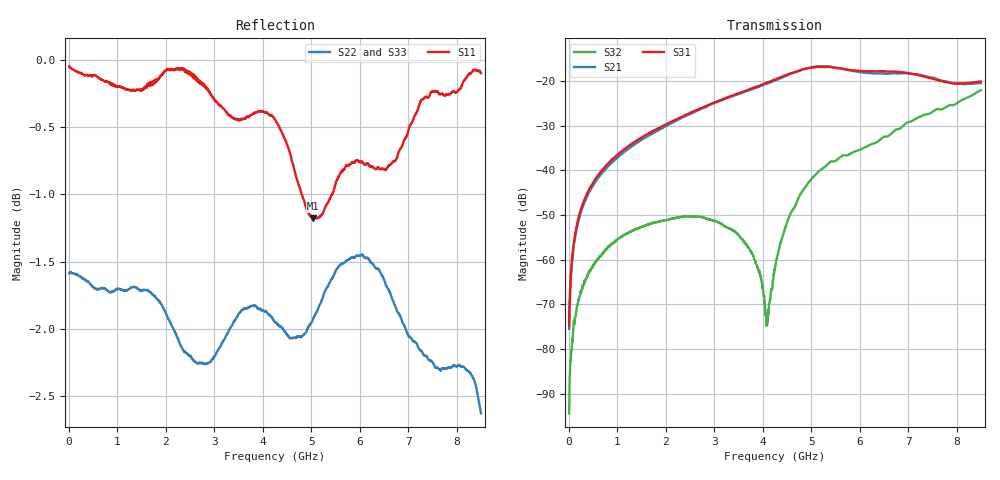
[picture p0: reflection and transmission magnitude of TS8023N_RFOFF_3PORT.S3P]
!Agilent Technologies,E5071C,MY46522130,B.12.04
!Date: Thu Jul 17 20:36:12 2025
!Data & Calibration Information:
!Freq	S11:SOLT3(ON)	S13:SOLT3(ON)	S14:SOLT3(ON)
!	S31:SOLT3(ON)	S33:SOLT3(ON)	S34:SOLT3(ON)
!	S41:SOLT3(ON)	S43:SOLT3(ON)	S44:SOLT3(ON)
!PortZ  Port1:50+j0  Port3:50+j0  Port4:50+j0
!Above PortZ is port z conversion or system Z0 setting when saving the data.
!When reading, reference impedance value at option line is always used.
# Hz S dB R 50
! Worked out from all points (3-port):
!   1601 points, 10 MHz to 8.5 GHz, reference 50 ohm
!   strongest paths, dB at 10 MHz, 2.132 GHz, 4.255 GHz, 6.378 GHz, 8.5 GHz:
!     S31: -74.8, -29.0, -19.6, -17.8, -20.1
!     S21: -75.4, -29.4, -19.9, -18.3, -20.5
!     S32: -94.4, -50.8, -61.7, -33.5, -22.0
!   lowest |S11| = -1.2 dB at 5.04 GHz (marker M1), VSWR 14.74, Z = 3.4 + j2.22 ohm
!   |S11| at or under -10 dB: nowhere
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1e7  -0.05 -0.5  -74.37 58.2  -75.07 60.6
     -75.45 56.6  -1.59 179.8  -91.99 101.7
     -74.82 56.5  -94.37 90.6  -1.72 179.8
2.063312e8  -0.09 -10.3  -51.17 87.2  -50.46 86.6
            -51.21 87.1  -1.61 177.9  -69.61 83.2
            -50.56 86.8  -68.85 87.4  -1.74 177.8
7.422625e8  -0.16 -33.6  -39.87 86.3  -39.22 85.1
            -39.94 86.4  -1.70 169.7  -58.00 82.2
            -39.26 85.3  -57.97 81.3  -1.87 169.7
3.029256e9  -0.31 -96.7  -24.78 65.1  -24.66 62.3
            -24.82 65.0  -2.19 122.7  -51.35 42.1
            -24.69 62.3  -51.40 42.7  -2.25 120.6
4.090506e9  -0.39 -129.6  -20.63 46.0  -20.37 42.9
            -20.59 45.2  -1.88 103.8  -74.08 103.8
            -20.33 42.3  -74.71 107.2  -2.12 101.5
4.255e9  -0.45 -135.5  -19.95 42.5  -19.70 38.9
         -19.85 42.2  -1.95 101.5  -61.83 -177.9
         -19.63 38.5  -61.73 -177.8  -2.19 97.8
5.040325e9  -1.18 174.9  -16.91 13.6  -17.03 9.3
            -16.82 13.8  -1.92 84.2  -41.52 163.6
            -16.95 9.4  -41.51 163.4  -1.88 78.6
5.963612e9  -0.75 108.5  -17.94 -19.8  -17.67 -22.5
            -17.94 -20.1  -1.46 77.0  -35.63 130.4
            -17.69 -22.8  -35.55 130.5  -1.66 77.2
7.253031e9  -0.31 57.1  -18.65 -46.2  -18.80 -53.7
            -18.61 -46.6  -2.16 71.1  -27.87 106.2
            -18.78 -53.7  -27.93 106.3  -2.04 59.0
8.5e9  -0.10 57.5  -20.41 -51.8  -20.07 -58.2
       -20.46 -51.6  -2.63 59.9  -22.02 87.7
       -20.10 -58.7  -22.04 87.2  -3.01 55.1
